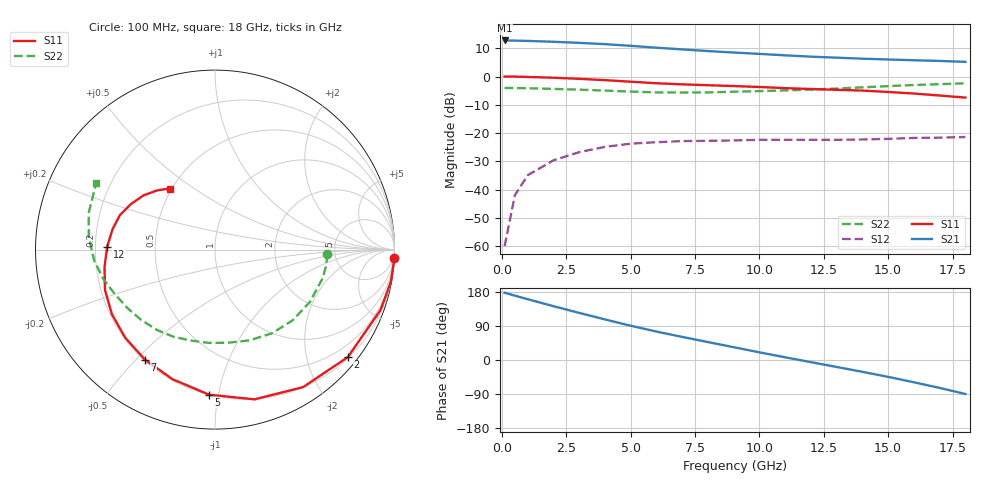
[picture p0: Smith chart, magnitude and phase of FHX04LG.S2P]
! SCCS file tdata/fujitsu: @(#)get -r1.1 /eesof/src/tdata/fujitsu/s.fhx04lg.s2p # Version date: 9/24/90
! FHX04LG.S2P  8/88
! FHX04/05/06FA/LG
! @2V-10mA
! .1GHZ 18GHZ 20
# GHZ S MA R 50
! S-parameter data
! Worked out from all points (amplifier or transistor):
!   20 points, 100 MHz to 18 GHz, reference 50 ohm
!   highest |S21| = 12.7 dB at 100 MHz (marker M1)
!   |S21| within 3 dB of that: start of sweep to 6.738 GHz
!   unconditionally stable (mu >= 1): 10.57 GHz to end of sweep
!   at 2 GHz: K = 0.26, MSG = 21.0 dB, |S12| = -29.6 dB
!   at 9 GHz: K = 0.90, MSG = 15.5 dB, |S12| = -22.6 dB
!   at 18 GHz: K = 1.18, MAG = 10.7 dB, |S12| = -21.4 dB
!   lowest NFmin = 0.33 dB at 2 GHz
!   S11 on the Smith chart (normalised r, x): 100 MHz: -1, -44; 2 GHz: 0.22, -2.81; 5 GHz: 0.20, -0.94; 7 GHz: 0.20, -0.53; 12 GHz: 0.25, +0.01; 18 GHz: 0.49, +0.40
0.1  1.001 -2.6  4.34 177.5  0.001 86.0  0.627 -2.3
0.5  0.996 -10.3  4.309 169.8  0.008 83.6  0.626 -8.1
1  0.982 -20.0  4.257 160.4  0.018 74.8  0.62 -15.2
2  0.952 -39.0  4.113 142.0  0.033 62.9  0.604 -28.9
3  0.91 -57.3  3.934 124.3  0.046 51.5  0.585 -42.4
4  0.863 -75.2  3.735 107.0  0.057 40.3  0.564 -55.8
5  0.809 -92.3  3.487 90.4  0.065 30.3  0.541 -69.2
6  0.76 -108.1  3.231 75.0  0.069 21.0  0.524 -82.0
7  0.727 -122.4  3.018 60.9  0.072 14.1  0.521 -93.6
8  0.701 -135.5  2.817 47.3  0.073 7.9  0.524 -104.7
9  0.678 -147.9  2.656 33.8  0.074 1.6  0.538 -115.4
10  0.653 -159.8  2.512 20.2  0.076 -4.0  0.552 -125.7
11  0.623 -171.1  2.367 7.1  0.076 -10.1  0.568 -136.4
12  0.601 178.5  2.245 -5.7  0.076 -15.9  0.587 -146.4
13  0.582 168.8  2.153 -18.4  0.076 -21.9  0.611 -156.2
14  0.564 160.2  2.065 -31.2  0.077 -28.6  0.644 -165.4
15  0.533 151.6  2.001 -44.5  0.079 -36.8  0.676 -174.8
16  0.5 142.8  1.938 -58.8  0.082 -48.5  0.707 174.2
17  0.461 134.3  1.884 -73.7  0.083 -61.7  0.733 163.6
18  0.424 126.6  1.817 -89.7  0.085 -77.9  0.758 150.9
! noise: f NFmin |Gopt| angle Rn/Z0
2  0.33  0.81  18  0.4
4  0.35  0.75  54  0.36
6  0.45  0.69  93  0.25
8  0.55  0.62  125  0.15
10  0.66  0.53  147  0.11
12  0.75  0.47  175  0.08
14  0.88  0.42  -157  0.08
16  1.15  0.36  -133  0.07
18  1.3  0.27  -105  0.07
